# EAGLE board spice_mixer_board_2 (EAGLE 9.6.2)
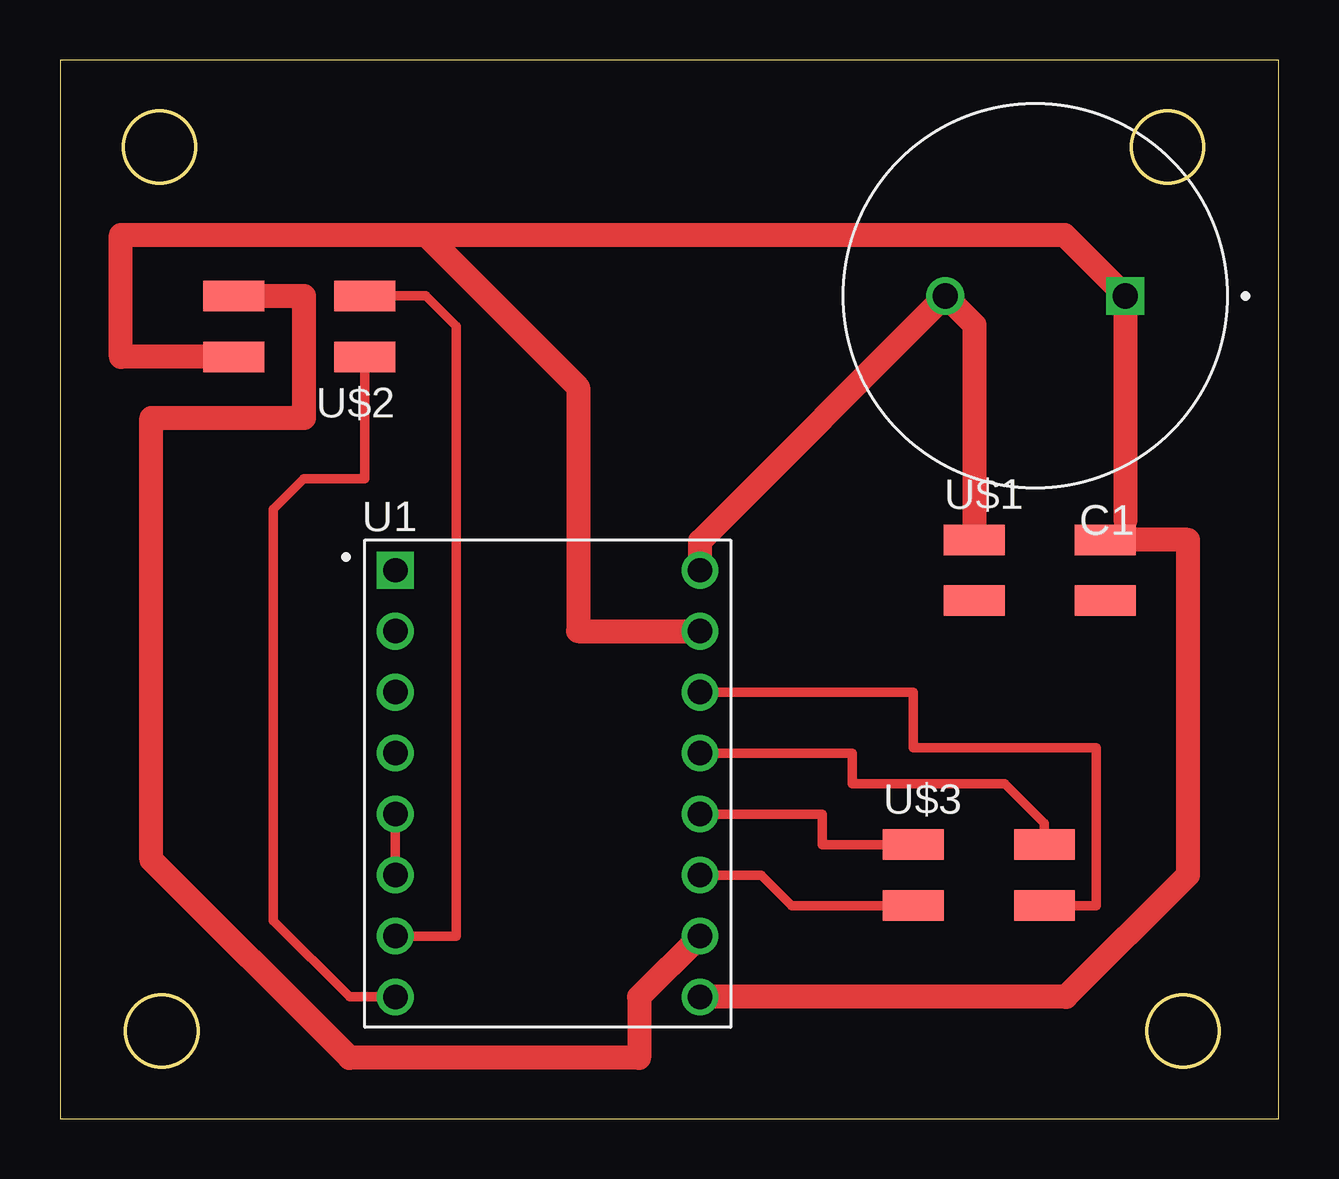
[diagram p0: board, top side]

Size 50.78 x 44.12 mm. Coordinates in mm from the lower left corner, seen from the top.
Outline: 0,0 50.78,0 50.78,44.12 0,44.12 0,0
Outline: circle at 4.15,40.49 radius 1.5
Outline: circle at 46.15,40.49 radius 1.5
Outline: circle at 46.78,3.66 radius 1.5
Outline: circle at 4.24,3.66 radius 1.5
Copper layers (1*16): Top 0.035mm / dielectric 1.5mm / Bottom 0.035mm
Design rules "default *": minimum track width 6mil, minimum drill 0.35mm, track to track 0.4mm, track to pad 0.4mm, pad to pad 0.4mm, via to via 0.4mm, smd to smd 0.4mm, copper to edge 40mil, drill to drill 6mil, minimum pad ring 10mil, minimum via ring 8mil, stop-mask expansion 4mil, vias tented up to drill 0mil, thermal gap 10mil
Net classes: 0 default: width 0.4 mm, clearance 0.4 mm; 1 MOTOR: width 0.4 mm, clearance 0.4 mm; 2 STEP: width 0.4 mm, clearance 0.4 mm; 3 VDD: width 0.4 mm, clearance 0.4 mm; 4 DIR: width 0.4 mm, clearance 0.4 mm; 5 GND: width 0.4 mm, clearance 0.4 mm

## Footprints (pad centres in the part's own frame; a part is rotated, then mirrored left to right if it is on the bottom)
CAPPRD750W80D1600H2000 = drill 1.05 pad 1.4: N 3.75,0 | drill 1.05 pad 1.4 square: P -3.75,0
MODULE_A4988_STEPPER_MOTOR_DRIVER_CARRIER = drill 1.02 square: 1 -6.35,8.89 | drill 1.02: 2 -6.35,6.35; 3 -6.35,3.81; 4 -6.35,1.27; 5 -6.35,-1.27; 6 -6.35,-3.81; 7 -6.35,-6.35; 8 -6.35,-8.89; 9 6.35,-8.89; 10 6.35,-6.35; 11 6.35,-3.81; 12 6.35,-1.27; 13 6.35,1.27; 14 6.35,3.81; 15 6.35,6.35; 16 6.35,8.89
2X02SMD = smd 2.54 x 1.27: 1 -2.54,1.27; 2 2.92,1.27; 3 -2.54,-1.27; 4 2.92,-1.27

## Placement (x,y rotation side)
C1  EEUFS1J681S  [CAPPRD750W80D1600H2000]  40.64,34.29 180 top
U1  A4988_STEPPER_MOTOR_DRIVER_CARRIER  [MODULE_A4988_STEPPER_MOTOR_DRIVER_CARRIER]  20.32,13.97 0 top
U$1  CONN_02X2-PINHEAD-SMD  [2X02SMD]  40.64,22.86 0 top
U$2  CONN_02X2-PINHEAD-SMD  [2X02SMD]  10.16,33.02 180 top
U$3  CONN_02X2-PINHEAD-SMD  [2X02SMD]  38.1,10.16 0 top

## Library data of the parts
C1 = EEUFS1J681S; AVAILABILITY: In Stock; DESCRIPTION: CAP ALUM 680UF 20% 63V THRU HOLE; MF: Panasonic; MP: EEUFS1J681S; PACKAGE: RADIAL-2 Panasonic; PRICE: None; PURCHASE-URL: https://pricing.snapeda.com/search/part/EEUFS1J681S/?ref=eda
U1 = A4988_STEPPER_MOTOR_DRIVER_CARRIER; AVAILABILITY: Not in stock; DESCRIPTION: Stepper Motor Driver; MF: Pololu; MP: A4988 STEPPER MOTOR DRIVER CARRIER; PACKAGE: None; PRICE: None
U$1-U$3 = fab-emma-re8nowiwt7yj8fhybscymuq61o

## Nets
GND [GND]: C1.P U1.9 U1.15 U$1.2 U$2.2
MOTOR [MOTOR]: C1.N U1.16 U$1.1
N$1: U1.13 U$3.2
N$3: U1.12 U$3.1
N$4: U1.11 U$3.3
N$5: U1.5 U1.6
N$6: U1.14 U$3.4
N$28: U1.8 U$2.1
N$29: U1.7 U$2.3
VDD [VDD]: U1.10 U$2.4

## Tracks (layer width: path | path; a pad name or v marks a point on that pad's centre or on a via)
GND
  Top 0.4: 44.39,24.96 U$1.2
  Top 1: U$2.2 2.54,31.75 2.54,36.83 15.24,36.83 | 15.24,36.83 21.59,30.48 21.59,20.32 U1.15 | 15.24,36.83 41.85,36.83 C1.P 44.39,24.96 | U$1.2 46.99,24.13 46.99,10.16 41.91,5.08 U1.9
MOTOR
  Top 1: U1.16 26.67,24.07 C1.N 38.1,33.08 U$1.1
N$1
  Top 0.4: U$3.2 41.02,12.32 39.37,13.97 33.02,13.97 33.02,15.24 U1.13
N$3
  Top 0.4: U1.12 31.75,12.7 31.75,11.43 U$3.1
N$4
  Top 0.4: U$3.3 30.48,8.89 29.21,10.16 U1.11
N$5
  Top 0.4: U1.6 U1.5
N$6
  Top 0.4: U1.14 35.56,17.78 35.56,15.47 43.18,15.47 43.18,8.89 U$3.4
N$28
  Top 0.4: U1.8 12.06,5.08 8.89,8.26 8.89,25.4 10.16,26.67 12.7,26.67 U$2.1
N$29
  Top 0.4: U$2.3 15.24,34.29 16.51,33.02 16.51,7.62 U1.7
VDD
  Top 1: U1.10 24.13,5.08 24.13,2.54 12.06,2.54 3.81,10.79 3.81,29.21 10.16,29.21 10.16,34.29 U$2.4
